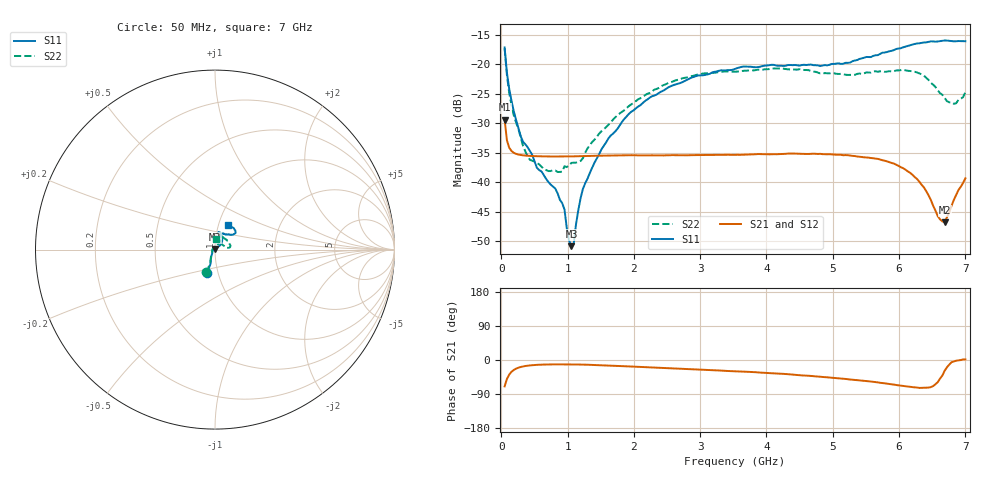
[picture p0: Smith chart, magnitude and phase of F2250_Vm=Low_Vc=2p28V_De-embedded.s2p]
! Integrated Device Technology
! Corporate Headquarters
! 6024 Silver Creek Valley Road
! San Jose, CA 95138  USA
! Phone:  1-408-284-8200
! Toll Free:  1-800-223-1366
! Webpage:  http://www.idt.com/
! Timing and RF Division
! 515 Groton Road, Suite 102
! Westford, MA 01886-6024
! Device:  F2250
! Description: Voltage Variable RF Attenuator
! Frequency:  50.0 -  6000.00 MHz
! Package:  3x3 mm Thin QFN Plastic Package: 16 pin
! Ports:  2 RF, 3 DC
!  Pin  1  = GND
!  Pin  2  = NC
!  Pin  3  = RF1  = Port 1
!  Pin  4  = NC
!  Pin  5  = GND
!  Pin  6  = GND
!  Pin  7  = GND
!  Pin  8  = GND
!  Pin  9  = NC
!  Pin 10  = RF2  = Port 2
!  Pin 11  = NC
!  Pin 12  = GND
!  Pin 13  = GND
!  Pin 14  = VCNTRL
!  Pin 15  = VDD
!  Pin 16  = VMODE
! Vcntrl:  2.280 Volts
! Vmode:  +0.000 Volts
! Vdd:  +3.30  Volts
! Current:  1.178 mA
! Data:  The device was measured on a the F2250 evaluation board which has
!  individual transmission lines to the RF pins.  Data was collected
!  using a calibrated network analyzer.  The evaluation board was
!  de-embedded using a TRL calibration technique.
!  The reference plane is the edge of the package pin.
! Misc:  SN 10
!  Action Tracker AT0258
! Date Measured:  2014-11-26
! Date:  2015-10-15  MJV
! Note:
!  Integrated Device Technology supplies this data as a sample of measured
!  data at the package pin for this product.  Your particular data for this
!  product may vary.
!  Data was taken at 25 degrees C.
!  Integrated Device Technology reserves the right to change this data at anytime.
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# GHz S dB R 50
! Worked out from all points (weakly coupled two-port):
!   201 points, 50 MHz to 7 GHz, reference 50 ohm
!   highest |S21| = -29.40 dB at 50 MHz (marker M1); lowest = -46.8 dB at 6.687 GHz (marker M2)
!   lowest |S11| = -50.8 dB at 1.058 GHz (marker M3), VSWR 1.01, Z = 49.8 + j0.238 ohm
!   |S11| at or under -10 dB: start of sweep to end of sweep
!   |S22| runs from -38.3 to -17.3 dB; largest |S21 - S12| = 6e-05
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0.05  -17.18 -108.6  -29.40 -69.6  -29.40 -69.6  -17.33 -110.7
0.08475  -21.45 -107.5  -32.89 -50.2  -32.89 -50.2  -21.83 -109.6
0.15425  -26.23 -116.5  -34.71 -31.0  -34.72 -31.0  -26.98 -121.2
0.29325  -32.21 -127.9  -35.39 -18.4  -35.39 -18.4  -32.42 -135.6
0.3975  -34.08 -141.8  -35.52 -15.0  -35.52 -15.0  -35.62 -158.9
0.5365  -37.54 -155.6  -35.59 -12.8  -35.59 -12.8  -36.75 178.4
0.91875  -43.54 158.0  -35.64 -11.5  -35.64 -11.5  -38.22 130.4
1.023  -49.91 143.9  -35.63 -11.6  -35.63 -11.6  -37.10 112.1
1.05775  -50.83 123.9  -35.63 -11.6  -35.63 -11.6  -36.73 106.9
1.0925  -50.45 89.3  -35.62 -11.7  -35.61 -11.7  -36.69 102.3
1.162  -44.70 57.1  -35.60 -11.9  -35.60 -11.9  -36.52 91.3
1.2315  -41.11 44.4  -35.57 -12.1  -35.57 -12.1  -35.93 81.8
1.6485  -32.11 42.1  -35.48 -14.7  -35.48 -14.7  -29.88 62.5
1.9265  -28.39 41.4  -35.43 -16.9  -35.42 -16.9  -27.08 55.2
2.37825  -24.87 47.4  -35.44 -20.4  -35.44 -20.4  -24.01 55.8
3.525  -20.80 72.5  -35.37 -29.6  -35.37 -29.6  -21.28 74.3
4.7065  -20.17 72.3  -35.17 -42.6  -35.17 -42.6  -21.25 72.0
5.85325  -17.81 40.5  -36.60 -63.3  -36.60 -63.3  -21.19 22.4
6.27025  -16.50 40.1  -39.44 -72.6  -39.44 -72.7  -21.41 9.1
6.68725  -15.99 48.8  -46.77 -28.4  -46.76 -28.0  -25.75 27.9
6.861  -16.13 55.1  -42.17 -1.8  -42.13 -1.8  -26.62 57.9
7  -16.12 63.2  -39.34 1.5  -39.30 1.3  -24.73 83.4
